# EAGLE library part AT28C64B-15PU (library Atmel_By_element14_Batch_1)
Parallel EEPROM
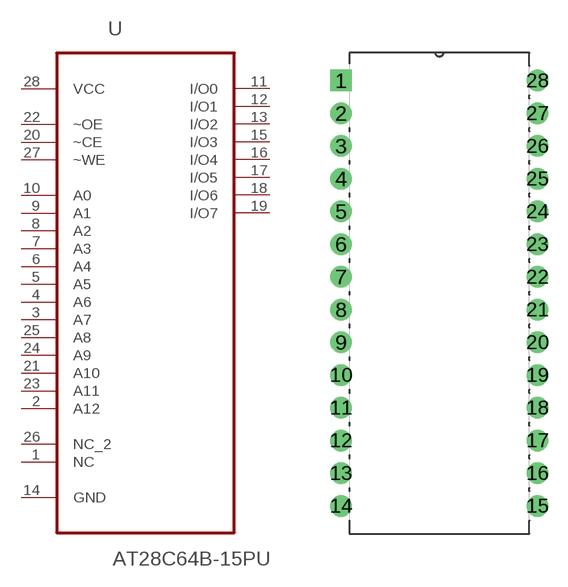
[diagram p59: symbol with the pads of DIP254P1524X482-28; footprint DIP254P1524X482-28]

Designator prefix U

## AT28C64B-15PU (DESCRIPTION: Parallel EEPROM; MPN: AT28C64B-15PU; OC_FARNELL: 1095784; OC_NEWARK: 96K6557; PACKAGE: PCDIP-28; SUPPLIER: ATMEL)  [DIP254P1524X482-28]
1  NC  nc
2  A12  in
3  A7  in
4  A6  in
5  A5  in
6  A4  in
7  A3  in
8  A2  in
9  A1  in
10  A0  in
11  I/O0  out
12  I/O1  out
13  I/O2  out
14  GND  pwr
15  I/O3  out
16  I/O4  out
17  I/O5  out
18  I/O6  out
19  I/O7  out
20  ~CE  in
21  A10  in
22  ~OE  pwr
23  A11  in
24  A9  in
25  A8  in
26  NC_2  nc
27  ~WE  in
28  VCC  pwr

## Footprint DIP254P1524X482-28 (pad centres in mm)
drill 1.118 square: 1 -15.24,33.02
drill 1.118: 2 -15.24,30.48; 3 -15.24,27.94; 4 -15.24,25.4; 5 -15.24,22.86; 6 -15.24,20.32; 7 -15.24,17.78; 8 -15.24,15.24; 9 -15.24,12.7; 10 -15.24,10.16; 11 -15.24,7.62; 12 -15.24,5.08; 13 -15.24,2.54; 14 -15.24,0; 15 0,0; 16 0,2.54; 17 0,5.08; 18 0,7.62; 19 0,10.16; 20 0,12.7; 21 0,15.24; 22 0,17.78; 23 0,20.32; 24 0,22.86; 25 0,25.4; 26 0,27.94; 27 0,30.48; 28 0,33.02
